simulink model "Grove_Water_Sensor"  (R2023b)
settings: Solver=ode1  StartTime=0.0  StopTime=60  FixedStep=0.001  RelTol=1e-3  EnableMultiTasking=on
libraries: arduinolib x4

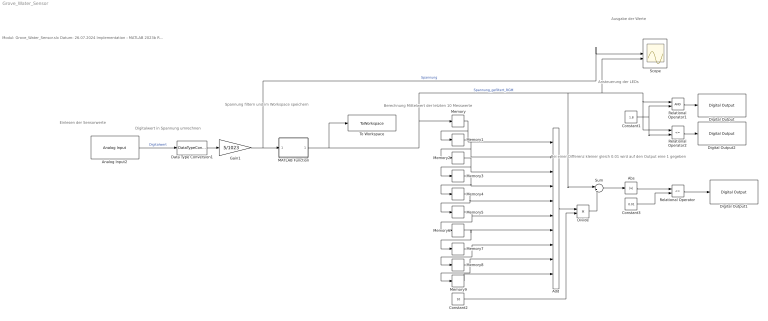
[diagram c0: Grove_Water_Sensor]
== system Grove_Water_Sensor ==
  note: Modul: Grove_Water_Sensor.slx Datum: 26.07.2024 Implementation : MATLAB 2023b Req. Toolbox : Simulink Support Package for Arduino Hardware Author : Denim Hilz Letzte Änderung : 25-07-2024
  note: Ansteuerung der LEDs
  note: Einlesen der Sensorwerte
  note: Ausgabe der Werte
  note: Digitalwert in Spannung umrechnen
  note: Bei einer Differenz kleiner gleich 0.01 wird auf den Output eine 1 gegeben
  note: Spannung filtern und im Workspace speichern
  note: Berechnung Mittelwert der letzten 10 Messwerte
  Abs : Abs
  Add : Sum  Inputs=++++++++++
  Analog Input2 : arduinolib/Analog Input  pinNumber=0  ReadResultsOnly=off  ConversionTriggerSource=Software  ExternalTriggerType=uint32( 0 )  OutputDataType=uint16  EnableConversionCompleteNotify=off  EnableOuputStatus=off  SampleTime=-1  blockPlatform=arduino
  Constant1 : Constant  Value=1.8
  Constant2 : Constant  Value=10
  Constant3 : Constant  Value=0.01
  Data Type Conversion1 : DataTypeConversion  OutDataTypeStr=double
  Digital Output : arduinolib/Digital Output  pinNumber=9  Direction=output  blockPlatform=arduino
  Digital Output1 : arduinolib/Digital Output  pinNumber=8  Direction=output  blockPlatform=arduino
  Digital Output2 : arduinolib/Digital Output  pinNumber=10  Direction=output  blockPlatform=arduino
  Divide : Product  Inputs=*/
  Gain1 : Gain  Gain=5/1023
  MATLAB Function : MATLAB Function  TreatAsAtomicUnit=on
  Memory{,1..9} (10 alike) : Memory
  Relational Operator : RelationalOperator  Operator=<=  OutDataTypeStr=boolean  RndMeth=Simplest
  Relational Operator1 : RelationalOperator  OutDataTypeStr=boolean  RndMeth=Simplest
  Relational Operator2 : RelationalOperator  Operator=<=  OutDataTypeStr=boolean  RndMeth=Simplest
  Scope : Scope  NumInputPorts=2
  Sum : Sum  Inputs=|+-
  To Workspace : ToWorkspace  VariableName=Spannung_gefiltert  SampleTime=-1
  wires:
  Analog Input2/1 -> Data Type Conversion1/1  "Digitalwert"
  MATLAB Function/1(RGM) -> To Workspace/1, Sum/1, Relational Operator2/1, Relational Operator1/1, Scope/2, Memory/1  "Spannung_gefiltert_RGM"
  Gain1/1 -> MATLAB Function/1(x), Scope/1  "Spannung"
  Data Type Conversion1/1 -> Gain1/1
  Memory/1 -> Memory1/1, Add/1
  Memory1/1 -> Memory2/1, Add/2
  Memory2/1 -> Memory3/1, Add/3
  Memory3/1 -> Memory4/1, Add/4
  Memory4/1 -> Memory5/1, Add/5
  Memory5/1 -> Memory6/1, Add/6
  Memory6/1 -> Memory7/1, Add/7
  Memory7/1 -> Memory8/1, Add/8
  Memory8/1 -> Memory9/1, Add/9
  Memory9/1 -> Add/10
  Constant2/1 -> Divide/2
  Add/1 -> Divide/1
  Divide/1 -> Sum/2
  Sum/1 -> Abs/1
  Abs/1 -> Relational Operator/1
  Constant3/1 -> Relational Operator/2
  Relational Operator/1 -> Digital Output1/1
  Relational Operator1/1 -> Digital Output/1
  Relational Operator2/1 -> Digital Output2/1
  Constant1/1 -> Relational Operator2/2, Relational Operator1/2

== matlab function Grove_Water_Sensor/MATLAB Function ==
function RGM = RekGleitenderMittelwert(x)

persistent n aSchieberegister
persistent bErsterDurchlauf

if isempty (bErsterDurchlauf)
    n = 80;
    aSchieberegister = x * ones (n,1);
    bErsterDurchlauf = 1;
end

for m=1:n-1
    aSchieberegister (m) = aSchieberegister(m+1);
end

aSchieberegister (n) = x;
RGM = x;

RGM = sum(aSchieberegister) / n;
end
